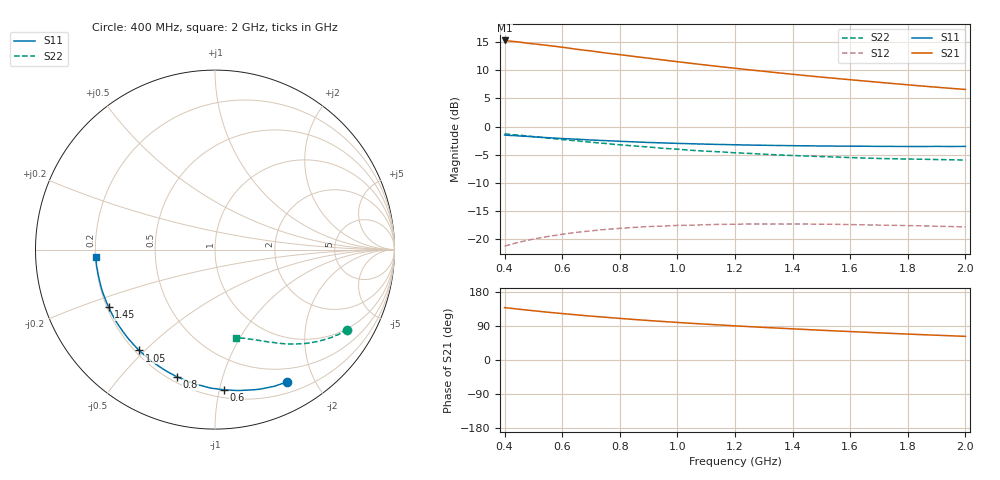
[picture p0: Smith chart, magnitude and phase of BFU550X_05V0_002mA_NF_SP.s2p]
! Filename:  P:\Prog\Test\Noise\ATS_data\Testdata_Net\BFU550X no attenuator noise\BFU550X_APG2013_44_C05_05p0V_002mA_NF_CM01_D.sf
! Date/Time: Fri 26/Jul/2013 14:37:11
! BFU550X_APG2013_44_C05_05p0V_1to10mA_NF_CM01_Bias2_R.sf
! Noise Parameter Data File
! BFU550X_APG2013_44_C05_05p0V_1to10mA_NF_CM01
! Date/time: Wed Jul 24 16:36:15 2013
! VAR V_out= 5.000000
! VAR I_out= 1.990000
! VAR V_in= 0.792900
! VAR I_in= 0.021605
! Device data file deembeded for feedlines and parallel
! Original file: \BFU550X no attenuator noise\BFU550X_APG2013_44_C05_05p0V_002mA_NF_CM01_R.sf
! Feed-files: PR005V01_100713_Feed1.s2p, PR005V01_100713_Feed2.s2p
! Parallel-file: PR005V01_100713_Par.s2p
# MHz S MA R 50
!  Freq-MHz  S11-mag  S11-arg  S21-mag  S21-arg  S12-mag  S12-arg  S22-mag  S22-arg
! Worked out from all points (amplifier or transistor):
!   37 points, 400 MHz to 2 GHz, reference 50 ohm
!   highest |S21| = 15.3 dB at 400 MHz (marker M1)
!   |S21| within 3 dB of that: start of sweep to 876 MHz
!   unconditionally stable (mu >= 1): nowhere
!   at 500 MHz: K = 0.16, MSG = 17.3 dB, |S12| = -20.0 dB
!   at 1.1 GHz: K = 0.33, MSG = 14.2 dB, |S12| = -17.4 dB
!   at 2 GHz: K = 0.63, MSG = 12.2 dB, |S12| = -17.8 dB
!   lowest NFmin = 0.55 dB at 420 MHz
!   S11 on the Smith chart (normalised r, x): 400 MHz: 0.32, -1.63; 600 MHz: 0.26, -1.03; 800 MHz: 0.23, -0.72; 1.05 GHz: 0.22, -0.48; 1.45 GHz: 0.21, -0.24; 2 GHz: 0.20, -0.03
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400  0.8398 -61.7  5.799 138.2  0.08681 54.6  0.8623 -31.1
420  0.8331 -64.3  5.718 136.5  0.08966 53.3  0.8496 -32.4
440  0.8287 -67.0  5.656 134.9  0.09271 52.0  0.8427 -33.4
500  0.8102 -74.6  5.415 130.0  0.1004 48.0  0.8143 -36.9
550  0.7958 -80.7  5.237 126.1  0.1057 44.9  0.7888 -39.5
600  0.7823 -86.5  5.054 122.5  0.1107 42.1  0.7667 -41.9
650  0.772 -91.7  4.845 119.1  0.1152 39.6  0.7466 -44.0
700  0.7591 -97.0  4.681 115.8  0.1187 37.1  0.725 -46.2
750  0.7493 -101.8  4.492 112.8  0.1221 34.9  0.7071 -47.9
800  0.7397 -106.6  4.341 109.8  0.1249 32.7  0.6883 -49.8
900  0.7218 -115.4  4.037 104.2  0.1296 28.9  0.6578 -53.0
950  0.7151 -119.4  3.894 101.6  0.1309 27.0  0.6411 -54.7
1050  0.7028 -126.9  3.63 96.8  0.1333 23.9  0.6149 -57.4
1100  0.6975 -130.4  3.506 94.5  0.1345 22.5  0.604 -58.6
1200  0.6885 -137.1  3.287 90.1  0.1358 19.8  0.5845 -61.1
1300  0.6818 -143.2  3.089 86.1  0.1363 17.4  0.5677 -63.4
1450  0.674 -151.5  2.823 80.3  0.1363 14.3  0.5469 -66.5
1500  0.6719 -154.2  2.743 78.5  0.1361 13.3  0.5412 -67.5
1600  0.6696 -159.2  2.6 75.0  0.1349 11.7  0.5304 -69.6
1750  0.6661 -166.0  2.404 70.0  0.1329 9.5  0.5178 -72.4
1850  0.6649 -170.2  2.286 66.9  0.1315 8.3  0.5127 -74.2
2000  0.6662 -176.2  2.131 62.4  0.1284 7.0  0.5045 -76.9
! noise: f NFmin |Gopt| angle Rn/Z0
400  0.596  0.4868  28.97  0.191
460  0.5527  0.4516  41.39  0.161
600  0.6623  0.4879  47.57  0.1885
800  0.6901  0.4542  65.61  0.1601
1000  0.7681  0.4628  81.96  0.1425
1200  0.8012  0.4714  97.45  0.1275
1400  0.921  0.4782  110  0.1199
1600  0.8749  0.4446  127.3  0.0881
1800  0.8791  0.5115  140.8  0.0643
2000  0.9652  0.5373  150.2  0.0603
